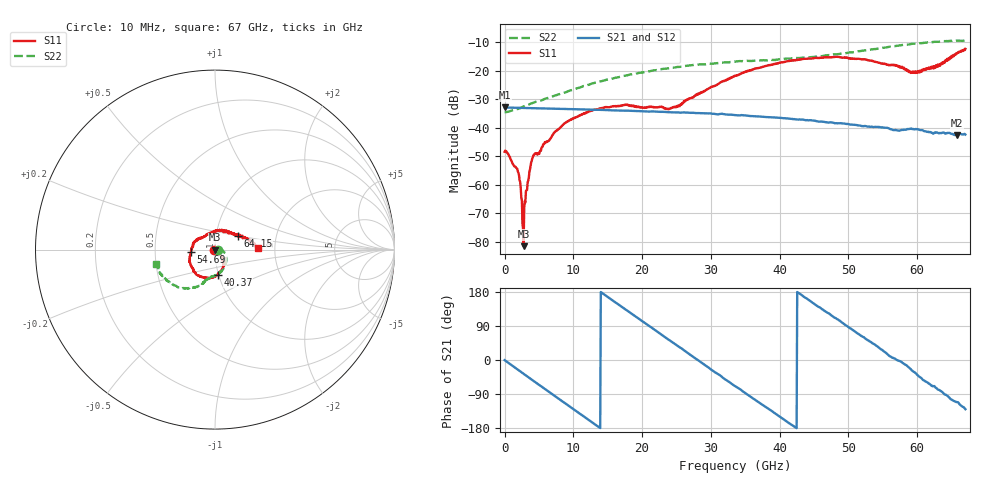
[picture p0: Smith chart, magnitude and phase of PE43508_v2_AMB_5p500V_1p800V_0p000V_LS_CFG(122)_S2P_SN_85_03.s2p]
!Keysight Technologies,N5227A,US51270237,A.10.43.00
!Date: Wednesday, August 22, 2018 17:19:26
!Correction: S11(Full 2 Port(1,3))
!S31(Full 2 Port(1,3))
!S13(Full 2 Port(1,3))
!S33(Full 2 Port(1,3))
!S2P File: Measurements: S11, S31, S13, S33:
# Hz S  dB  R 50
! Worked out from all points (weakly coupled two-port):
!   801 points, 10 MHz to 67 GHz, reference 50 ohm
!   highest |S21| = -32.89 dB at 10 MHz (marker M1); lowest = -42.6 dB at 65.74 GHz (marker M2)
!   lowest |S11| = -81.5 dB at 2.773 GHz (marker M3), VSWR 1.00, Z = 50 - j0.00673 ohm
!   |S11| at or under -10 dB: start of sweep to end of sweep
!   |S22| runs from -34.6 to -9.4 dB; largest |S21 - S12| = 0.00017
!   S11 on the Smith chart (normalised r, x): 10 MHz: 0.99, -0.00; 40.37 GHz: 0.99, -0.28; 54.69 GHz: 0.76, -0.02; 64.15 GHz: 1.27, +0.19; 67 GHz: 1.63, +0.03
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1e7  -48.41 -175.3  -32.89 -0.3  -32.90 -0.2  -34.59 -0.6
1.935962e9  -55.36 162.3  -33.04 -25.7  -33.04 -25.7  -33.43 6.6
2.187175e9  -58.44 172.2  -33.05 -29.0  -33.05 -29.0  -33.22 6.4
2.438388e9  -64.44 -170.5  -33.07 -32.3  -33.07 -32.3  -32.93 6.3
2.773338e9  -81.48 -53.0  -33.09 -36.6  -33.09 -36.6  -32.55 6.9
2.940812e9  -65.75 -13.6  -33.10 -38.8  -33.10 -38.8  -32.37 7.1
3.69445e9  -54.68 -37.8  -33.14 -48.5  -33.15 -48.6  -31.72 6.2
4.280612e9  -49.41 -27.2  -33.17 -56.0  -33.17 -56.1  -31.13 5.8
8.634962e9  -38.67 -60.6  -33.42 -112.0  -33.42 -112.0  -27.78 -4.6
1.123082e10  -35.28 -68.5  -33.58 -145.3  -33.58 -145.3  -25.63 -14.9
1.74274e10  -32.07 -87.6  -34.00 135.6  -34.00 135.6  -21.82 -39.0
2.236791e10  -32.75 -82.0  -34.43 72.5  -34.43 72.5  -19.72 -57.3
2.513125e10  -32.32 -64.4  -34.67 37.7  -34.66 37.7  -18.70 -66.1
3.3505e10  -21.89 -55.9  -35.58 -69.0  -35.58 -69.0  -16.83 -89.1
4.037148e10  -17.06 -83.5  -36.61 -154.0  -36.62 -154.1  -15.94 -100.6
4.472582e10  -15.74 -106.7  -37.47 151.8  -37.44 151.9  -15.28 -105.2
5.469059e10  -17.48 -174.8  -39.87 28.7  -39.84 28.4  -12.12 -120.9
5.586291e10  -18.16 171.5  -40.22 11.7  -40.20 11.3  -11.68 -124.2
5.979858e10  -20.33 113.3  -40.43 -35.0  -40.47 -35.5  -10.59 -136.3
6.415292e10  -16.66 30.3  -42.03 -91.4  -42.06 -91.9  -9.69 -153.2
6.574394e10  -14.10 13.7  -42.58 -111.1  -42.69 -111.4  -9.53 -159.8
6.7e10  -12.37 1.8  -42.39 -129.9  -42.44 -129.7  -9.45 -166.0
